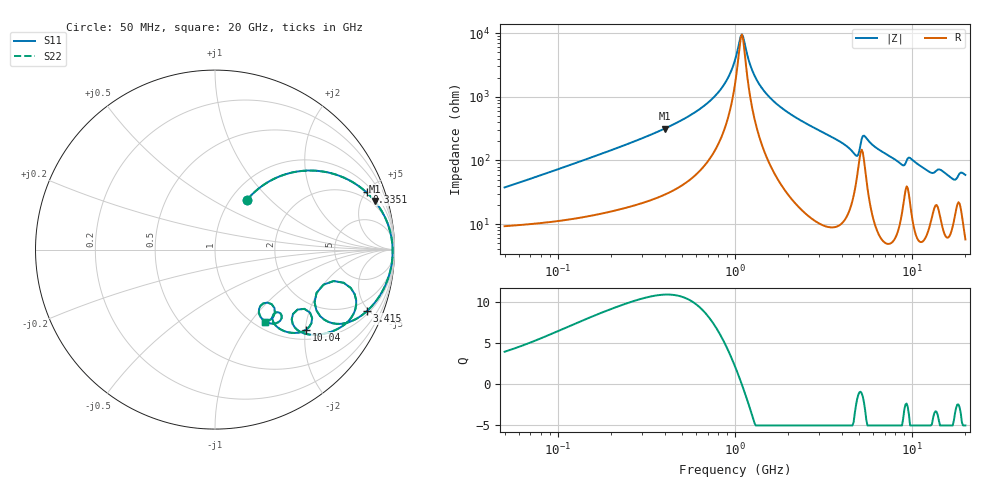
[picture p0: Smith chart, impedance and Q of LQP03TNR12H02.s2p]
!Murata Part Number: LQP03TNR12H02
!These Parameters are Measured in Series Mode Connection
!  o--[Z]--o
!Port1  Port2
!  o-------o
!Freq. Start=50[MHz] Stop=20[GHz], 401[Steps]
# Hz S RI R 50
!Freq.(Hz) S11(Real) S11(Imag) S21(Real) S21(Imag) S12(Real) S12(Imag) S22(Real) S22(Imag)
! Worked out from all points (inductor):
!   401 points, 50 MHz to 20 GHz, reference 50 ohm
!   read as one part in series: L = 115 nH near 51.52 MHz
!   highest Q = 10.9 at 401 MHz (marker M1), where L = 125 nH
!   self-resonance near 1.078 GHz
!   S11 on the Smith chart (normalised r, x): 50 MHz: 1.19, +0.73; 335.1 MHz: 1.48, +5.06; 3.415 GHz: 1.18, -4.88; 10.04 GHz: 1.24, -2.03; 20 GHz: 1.11, -1.18
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5e7  0.1766 0.2751  0.8234 -0.2751  0.8234 -0.2751  0.1766 0.2751
1.364002e8  0.4936 0.4392  0.5064 -0.4392  0.5064 -0.4392  0.4936 0.4392
3.350611e8  0.8442 0.3188  0.1558 -0.3188  0.1558 -0.3188  0.8442 0.3188
3.721004e8  0.8715 0.2916  0.1285 -0.2916  0.1285 -0.2916  0.8715 0.2916
4.010383e8  0.889 0.2715  0.111 -0.2715  0.111 -0.2715  0.889 0.2715
7.411344e8  0.9751 0.1034  0.0249 -0.1034  0.0249 -0.1034  0.9751 0.1034
8.870719e8  0.985 0.0553  0.015 -0.0553  0.015 -0.0553  0.985 0.0553
1e9  0.9885 0.0235  0.0115 -0.0235  0.0115 -0.0235  0.9885 0.0235
1.094034e9  0.9896 -0.000457  0.0104 0.000457  0.0104 0.000457  0.9896 -0.000457
1.251922e9  0.989 -0.0366  0.011 0.0366  0.011 0.0366  0.989 -0.0366
1.454215e9  0.9847 -0.0775  0.0153 0.0775  0.0153 0.0775  0.9847 -0.0775
2.728004e9  0.9118 -0.2664  0.0882 0.2664  0.0882 0.2664  0.9118 -0.2664
3.415248e9  0.8476 -0.3416  0.1524 0.3416  0.1524 0.3416  0.8476 -0.3416
4.748272e9  0.5854 -0.3701  0.4146 0.3701  0.4146 0.3701  0.5854 -0.3701
5.194772e9  0.7166 -0.1847  0.2834 0.1847  0.2834 0.1847  0.7166 -0.1847
5.598765e9  0.7812 -0.3347  0.2188 0.3347  0.2188 0.3347  0.7812 -0.3347
7.442007e9  0.5773 -0.4736  0.4227 0.4736  0.4227 0.4736  0.5773 -0.4736
8.774992e9  0.4328 -0.4142  0.5672 0.4142  0.5672 0.4142  0.4328 -0.4142
1.004137e10  0.5092 -0.4452  0.4908 0.4452  0.4908 0.4452  0.5092 -0.4452
1.257102e10  0.3244 -0.4024  0.6756 0.4024  0.6756 0.4024  0.3244 -0.4024
1.800918e10  0.2911 -0.295  0.7089 0.295  0.7089 0.295  0.2911 -0.295
2e10  0.2782 -0.4021  0.7218 0.4021  0.7218 0.4021  0.2782 -0.4021
